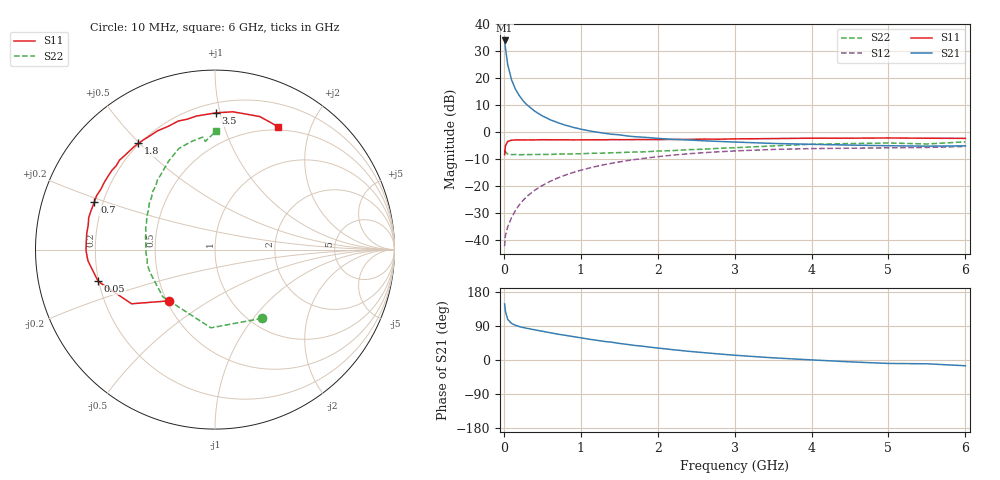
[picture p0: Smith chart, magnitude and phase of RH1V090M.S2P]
! SIEMENS Small Signal Semiconductors
! BFR106
! Si NPN RF Bipolar Junction Transistor in SOT23
! VCE = 1 V  IC = 90 mA
! Common Emitter S-Parameters:  August  1996
# GHz  S  MA  R  50
!  f  S11  S21  S12  S22
! GHz  MAG  ANG  MAG  ANG  MAG  ANG  MAG  ANG
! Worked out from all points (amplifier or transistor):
!   36 points, 10 MHz to 6 GHz, reference 50 ohm
!   highest |S21| = 34.0 dB at 10 MHz (marker M1)
!   |S21| within 3 dB of that: start of sweep to 21.59 MHz
!   unconditionally stable (mu >= 1): 60.94 MHz to end of sweep
!   at 250 MHz: K = 1.34, MAG = 15.0 dB, |S12| = -25.3 dB
!   at 1.4 GHz: K = 1.21, MAG = 2.6 dB, |S12| = -11.5 dB
!   at 6 GHz: K = 1.04, MAG = -1.1 dB, |S12| = -5.3 dB
!   S11 on the Smith chart (normalised r, x): 10 MHz: 0.51, -0.34; 50 MHz: 0.20, -0.13; 700 MHz: 0.17, +0.19; 1.8 GHz: 0.20, +0.50; 3.5 GHz: 0.27, +0.97; 6 GHz: 0.46, +1.54
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0.01  0.3831 -131.8  50.29 147.9  0.0077 60.1  0.464 -55.6
0.02  0.5541 -147.0  36.98 129.0  0.0121 52.6  0.4363 -93.0
0.05  0.6746 -164.8  18.02 107.2  0.0176 51.5  0.3919 -137.9
0.1  0.7108 -175.0  9.372 96.5  0.026 60.5  0.3833 -159.9
0.15  0.7185 -179.5  6.328 91.7  0.0352 65.4  0.3869 -167.5
0.2  0.7187 177.3  4.786 88.3  0.0449 68.7  0.3814 -172.1
0.25  0.7185 175.3  3.83 85.7  0.0545 70.0  0.3838 -175.7
0.3  0.7203 173.0  3.226 83.7  0.0644 70.8  0.3849 -177.5
0.4  0.7194 169.1  2.466 79.6  0.0838 70.8  0.3858 178.8
0.5  0.7261 165.7  2.007 75.9  0.1027 70.4  0.3869 175.8
0.6  0.7237 162.2  1.71 72.0  0.1223 69.1  0.387 173.6
0.7  0.7223 158.4  1.506 68.3  0.1415 67.8  0.3914 171.4
0.9  0.7195 152.2  1.233 61.8  0.179 64.3  0.395 166.6
1.1  0.7228 145.5  1.067 55.2  0.2145 60.7  0.4042 163.0
1.3  0.7219 139.7  0.96 49.2  0.2488 56.6  0.4098 158.6
1.8  0.73 125.8  0.809 36.4  0.3248 46.7  0.4313 148.9
2.2  0.735 115.9  0.736 27.2  0.3762 39.1  0.4564 141.0
3.5  0.7619 89.6  0.619 5.7  0.4791 16.9  0.557 117.6
4.5  0.775 76.6  0.577 -4.9  0.5047 3.5  0.616 102.5
5  0.7821 71.4  0.561 -9.1  0.5129 -1.8  0.6307 96.2
5.5  0.773 66.4  0.551 -10.0  0.5218 -4.1  0.6055 95.1
6  0.7691 62.8  0.559 -15.2  0.5422 -10.4  0.6623 89.3
